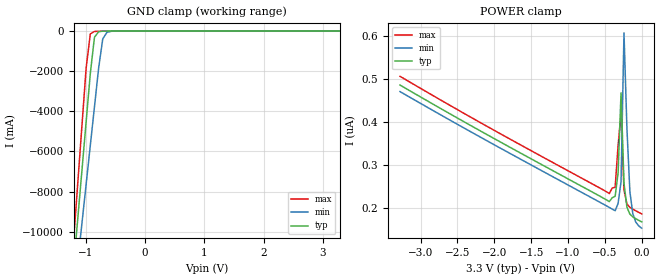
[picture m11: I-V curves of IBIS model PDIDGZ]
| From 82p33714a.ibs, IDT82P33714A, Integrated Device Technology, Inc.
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|   Model PDIDGZ
[Model]  PDIDGZ
Model_type Input
Polarity   Non-Inverting
Vinl =   0.8000V
Vinh =   2.0000V
C_comp   2.6812pF   2.6701pF   2.6826pF
[Temperature Range]   25.0000   0.1250k   -40.0000
[Voltage Range]   3.3000V   3.0000V   3.6000V
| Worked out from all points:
|   GND clamp passes 1 mA (typ) near -0.64 V on its own axis
[GND_clamp]
|Voltage   I(typ)   I(min)   I(max)
-3.3V     -83.46A    -71.04A    -95.7A
-1.2V     -11.69A    -13.39A    -10.37A
-1.13V    -9.3A      -11.47A    -7.522A
-1.06V    -6.904A    -9.549A    -4.675A
-990mV    -4.509A    -7.624A    -1.828A
-920mV    -2.113A    -5.699A    -140.7mA
-850mV    -308.3mA   -3.775A    -17.61mA
-780mV    -30.18mA   -1.85A     -8.684mA
-710mV    -4.231mA   -388.3mA   -4.536mA
-640mV    -826.8uA   -62.95mA   -1.713mA
-430mV    -4.377uA   -246.1uA   -5.398uA
3.28V     165.3nA    260.6nA    156.9nA
[POWER_clamp]
|Voltage   I(typ)   I(min)   I(max)
-3.28V    486.2nA    470.9nA    506.6nA
-440mV    214.3nA    200.8nA    233.1nA
-400mV    223.3nA    196.9nA    246nA
-360mV    226.7nA    193.1nA    247.8nA
-320mV    280.6nA    210nA      345.3nA
-280mV    468.1nA    260.6nA    421.2nA
-240mV    257.3nA    607.9nA    241nA
-200mV    201.3nA    384.8nA    208.8nA
-160mV    185.2nA    237.6nA    200.8nA
-120mV    178.7nA    185.9nA    196.6nA
-80mV     174.4nA    166.5nA    192.9nA
0V        167.1nA    152.4nA    185.7nA
